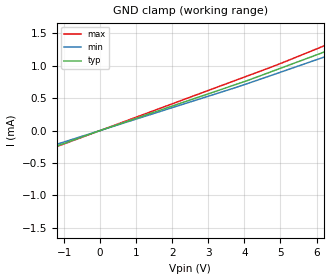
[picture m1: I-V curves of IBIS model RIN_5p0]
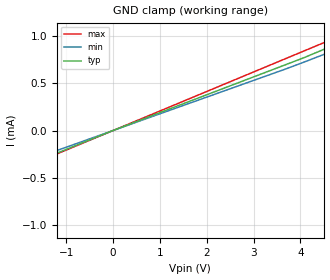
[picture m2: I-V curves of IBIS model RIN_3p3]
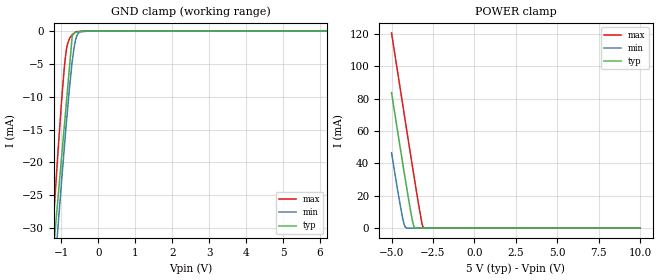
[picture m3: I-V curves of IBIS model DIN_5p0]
| TEXAS INSTRUMENTS INCORPORATED
| Standard Linear and Logic Group
| IBIS Model of TRS3232E RGT
| 3-V TO 5.5-V MULTICHANNEL RS-232 LINE DRIVER/RECEIVER WITH +/-15-kV IEC
| ESD PROTECTION
| This file contains package information for the following:
| VQFN - 16-pin (RGT) package as [Component] TRS3232E RGT
| This device can be powered at the following Vccs:
|  5 volt Vcc
|  3.3 volt Vcc
| This file provides unique models under the [Model Selector] for each Vcc.
| For operation at a specific Vcc, select the appropriate model after each
| [Model Selector] keyword.
| DOUT Models : DOUT buffer works on VPLUS and VMINUS Supply rails
|   (Chargepump Output Voltage).
|   - DOUT_5p0 Model captures the corresponding chargepump and
|   transient response of the bufer when VCC = 5V
|   - DOUT_3p3 Model captures the corresponding chargepump and
|   transient response of the bufer when VCC = 3.3V
[IBIS Ver]   3.2
[Comment char]  |_char
[File Name]   trs3232e_rgt.ibs
[File Rev]   1.0 | x_die
[Date]   October 29, 2020
[Source]   Data created from TI-SPICE simulations at TI-SLL.
[Notes]   The following is an IBIS list for TRS3232E RGT
[Disclaimer] Property of Texas Instruments Incorporated.  Unauthorized
   reproduction and/or distribution is strictly prohibited.
   This product is protected under copyright law.
   Created  2020, (C) Copyright  2020, Texas Instruments
   Incorporated, All Rights Reserved
   UNLESS THERE IS A SIGNED, WRITTEN AGREEMENT TO THE
   CONTRARY, TEXAS INSTRUMENTS (TI) IS PROVIDING THE IBIS
   MODELS  AND WITHOUT ANY WARRANTY, EXPRESSED OR
   IMPLIED.  TI assumes no liability for:
   1) the accuracy of the IBIS models provided to your
   company;
   2) the proper functioning of these IBIS Models in your
   design or for any resulting applications; or
   3) infringement of patents, copyrights or intellectual
   property rights resulting from your use of these IBIS
   models.
   TI provides IBIS Models as a service to our customers.
   You and your company shall not distribute, sell or give
   these models to anyone else without prior written
   permission from TI.
   TI reserves the right to make changes to our products or
   to discontinue any semiconductor product or service
   without notice, and advises our customers to obtain the
   latest version of relevant information to verify, before
   placing orders, that the information being relied on is
   current.
   Please be aware that your receipt and use of the IBIS
   information provided shall serve as acceptance of these
   terms and conditions.  If you do not accept these terms,
   you should return or destroy the IBIS models and any
   other accompanying information immediately.
| Component TRS3232E RGT
[Component]   TRS3232E_RGT
[Manufacturer]   Texas Instruments, Inc.
[Package]   |QFN (RGT) 16-pin
|   typ   min   max
R_pkg   0.0658   0.0248   0.0806
L_pkg   0.8404nH   0.6985nH   1.0659nH
C_pkg   0.1111pF   0.1026pF   0.1480pF
[Pin]   signal_name   model_name   R_pin   L_pin   C_pin
1   C1P   NC   na   na   na
2   VPLUS   POWER   na   na   na
3   C1N   NC   na   na   na
4   C2P   NC   na   na   na
5   C2N   NC   na   na   na
6   VMINUS   POWER   na   na   na
7   DOUT2   DOUT   na   na   na
8   RIN2   RIN   na   na   na
9   ROUT2   ROUT   na   na   na
10   DIN2   DIN   na   na   na
11   DIN1   DIN   na   na   na
12   ROUT1   ROUT   na   na   na
13   RIN1   RIN   na   na   na
14   DOUT1   DOUT   na   na   na
15   GND   GND   na   na   na
16   VCC   POWER   na   na   na
| Model RIN
[Model Selector]   RIN
RIN_5p0   5 volt Vcc
RIN_3p3   3.3 volt Vcc
| Model DIN
[Model Selector]   DIN
DIN_5p0   5 volt Vcc
DIN_3p3   3.3 volt Vcc
| Model ROUT
[Model Selector]   ROUT
ROUT_5p0   5 volt Vcc
ROUT_3p3   3.3 volt Vcc
| Model DOUT
[Model Selector]   DOUT
DOUT_5p0   5 volt Vcc
DOUT_3p3   3.3 volt Vcc
| Models and submodels in the file (8): RIN_5p0 (Input), RIN_3p3 (Input), DIN_5p0 (Input), DIN_3p3 (Input), ROUT_5p0 (3-state), ROUT_3p3 (3-state), DOUT_5p0 (3-state), DOUT_3p3 (3-state)
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[Model]   RIN_5p0
Model_type   Input
Vinl = 0.8
Vinh = 2.4
|   typ   min   max
C_comp   1.05pF   0.83pF   1.39pF
[Voltage Range]   5   4.5   5.5
[Temperature Range]   27   110   -40
[Power Clamp Reference]   5   4.5   5.5
[GND Clamp Reference]   0   0   0
[GND Clamp]
|   Voltage   I(typ)   I(min)   I(max)
-25V      -5.173mA   -4.828mA   -5.656mA
-11.64V   -2.393mA   -2.232mA   -2.618mA
-6.641V   -1.353mA   -1.262mA   -1.481mA
-3.141V   -625.6uA   -582.6uA   -685.6uA
-1.264V   -251.4uA   -222.5uA   -260.8uA
-43.29mV  -8.06uA    -7.513uA   -8.819uA
3.746V    705.9uA    660.3uA    771.1uA
4.874V    932.7uA    873.7uA    1.004mA
6.752V    1.32mA     1.236mA    1.427mA
8.416V    1.664mA    1.558mA    1.804mA
8.713V    1.725mA    1.616mA    1.871mA
25V       5.106mA    4.777mA    5.57mA
[Model]   RIN_3p3
Model_type   Input
Vinl = 0.6
Vinh = 2.4
|   typ   min   max
C_comp   1.07pF   0.83pF   1.45pF
[Voltage Range]   3.3   3   3.6
[Temperature Range]   27   110   -40
[Power Clamp Reference]   3.3   3   3.6
[GND Clamp Reference]   0   0   0
[GND Clamp]
|   Voltage   I(typ)   I(min)   I(max)
-25V      -5.173mA   -4.828mA   -5.656mA
-6.641V   -1.353mA   -1.262mA   -1.481mA
-3.868V   -776.6uA   -723.4uA   -850.7uA
-1.186V   -235.8uA   -208.5uA   -243.9uA
-43.29mV  -8.06uA    -7.513uA   -8.819uA
3.622V    682.5uA    637.9uA    745.6uA
5.203V    1.001mA    937uA      1.077mA
5.511V    1.064mA    996.4uA    1.146mA
5.88V     1.14mA     1.067mA    1.23mA
6.108V    1.187mA    1.112mA    1.281mA
25V       5.106mA    4.777mA    5.57mA
[Model]   DIN_5p0
Model_type   Input
Vinl = 0.8
Vinh = 2.4
|   typ   min   max
C_comp   0.75pF   0.72pF   0.79pF
[Voltage Range]   5   4.5   5.5
[Temperature Range]   27   110   -40
[Power Clamp Reference]   5   4.5   5.5
[GND Clamp Reference]   0   0   0
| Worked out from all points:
|   GND clamp passes 1 mA (typ) near -0.71 V on its own axis
|   POWER clamp passes 1 mA (typ) near -3.64 V on its own axis
[GND Clamp]
|   Voltage   I(typ)   I(min)   I(max)
-5V       -353.7mA   -333.1mA   -374.3mA
-1.343V   -44.3mA    -48.78mA   -40.41mA
-1.219V   -34.23mA   -39.59mA   -29.6mA
-1.161V   -30.19mA   -35.23mA   -24.64mA
-1.069V   -24.33mA   -28.57mA   -16.92mA
-884.1mV  -12.43mA   -15.57mA   -3.834mA
-824.5mV  -8.612mA   -11.7mA    -1.87mA
-702.6mV  -786.6uA   -4.649mA   -549.9uA
-611.8mV  -189.5uA   -1.343mA   -150.9uA
-513.5mV  -98.53uA   -211.2uA   -55.81uA
-284.9mV  -2.302uA   -935.4nA   -369.7nA
10V       0A         0A         0A
[POWER Clamp]
|   Voltage   I(typ)   I(min)   I(max)
-5V       83.65mA    46.54mA    120.6mA
-4.452V   48.08mA    12.84mA    84.53mA
-4.334V   40.54mA    6.495mA    76.82mA
-4.221V   33.3mA     1.772mA    69.38mA
-4.113V   26.49mA    140.8uA    62.32mA
-3.842V   10.11mA    164.9nA    44.74mA
-3.654V   1.221mA    38.71nA    32.63mA
-3.565V   74.33uA    0A         26.92mA
-3.242V   129.3nA    0A         7.188mA
-3.129V   0A         0A         1.622mA
-3.071V   0A         0A         250.9uA
10V       0A         0A         0A
